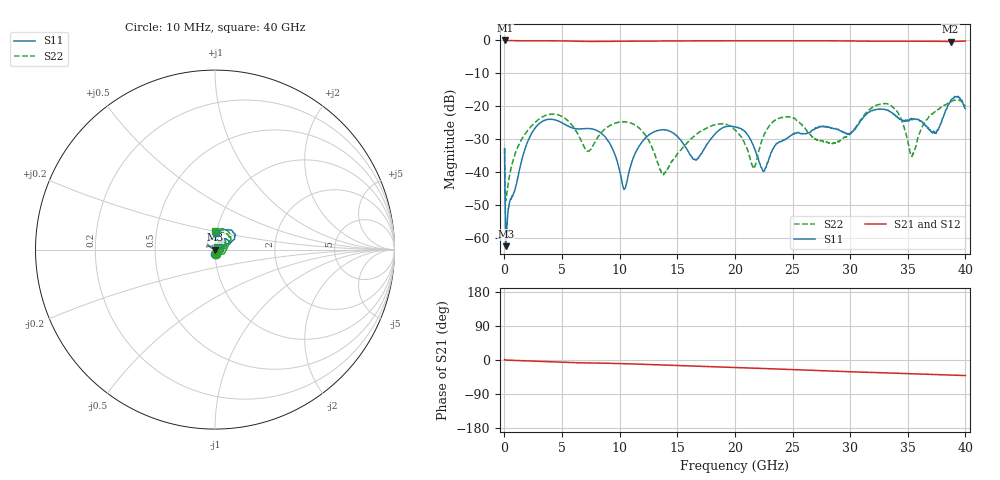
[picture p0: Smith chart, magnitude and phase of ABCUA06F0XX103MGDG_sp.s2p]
! Amotech Co.,Ltd.
! http://www.amotech.co.kr/
! Date: Wednesday, December 02, 2020 16:14:27
! Part Number: ABCUA 06F 0XX 103M GDG
! Freq. Start=10[MHz] Stop=40[GHz], 4000[Steps]
# Hz S  dB  R 50
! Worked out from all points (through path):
!   4000 points, 10 MHz to 40 GHz, reference 50 ohm
!   highest |S21| = -0.01 dB at 50 MHz (marker M1); lowest = -0.3 dB at 38.71 GHz (marker M2)
!   group delay of S21, straight-line fit = 2.85 ps
!   lowest |S11| = -62.4 dB at 140 MHz (marker M3), VSWR 1.00, Z = 49.9 + j0.0169 ohm
!   |S11| at or under -10 dB: start of sweep to end of sweep
!   |S22| runs from -48.5 to -18.0 dB; largest |S21 - S12| = 0.0046
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1e7  -32.76 -90.3  -0.02 1.3  -0.01 1.3  -32.72 -80.0
5e7  -47.88 -103.0  -0.01 0.2  -0.01 0.2  -45.68 -48.5
1.4e8  -62.35 167.2  -0.02 -0.2  -0.01 -0.2  -48.07 2.6
2.8e8  -52.97 97.8  -0.03 -0.5  -0.02 -0.5  -44.24 21.3
1.2e9  -40.93 145.3  -0.10 -1.6  -0.09 -1.5  -31.95 5.9
2.9e9  -25.57 142.3  -0.12 -3.2  -0.10 -3.2  -24.11 23.9
6.68e9  -26.78 22.5  -0.26 -7.4  -0.25 -7.4  -30.60 50.9
8.9e9  -29.97 -42.6  -0.29 -8.5  -0.27 -8.5  -26.33 -32.2
1.041e10  -44.95 -1.6  -0.23 -9.7  -0.22 -9.7  -24.69 -6.1
1.334e10  -27.29 -6.1  -0.15 -12.7  -0.13 -12.7  -37.41 104.8
1.655e10  -36.11 7.3  -0.13 -16.2  -0.11 -16.1  -28.82 -9.6
2.001e10  -26.24 31.6  -0.12 -19.8  -0.09 -19.7  -27.12 66.2
2.162e10  -32.12 17.7  -0.10 -21.5  -0.08 -21.4  -38.84 25.9
2.248e10  -39.57 56.3  -0.11 -22.5  -0.08 -22.4  -29.00 -23.0
2.452e10  -29.67 69.1  -0.11 -24.7  -0.09 -24.6  -23.15 18.4
2.667e10  -27.27 13.0  -0.11 -27.1  -0.09 -27.0  -29.05 65.2
2.888e10  -27.00 3.1  -0.14 -29.6  -0.11 -29.5  -30.75 47.4
3.334e10  -21.25 22.9  -0.24 -34.3  -0.22 -34.2  -19.41 61.9
3.538e10  -24.08 17.9  -0.24 -36.1  -0.22 -36.0  -35.09 41.5
3.734e10  -28.08 42.2  -0.26 -38.3  -0.24 -38.2  -21.65 20.1
3.871e10  -18.35 27.8  -0.34 -39.7  -0.31 -39.6  -18.60 43.7
4e10  -20.69 87.4  -0.19 -41.0  -0.17 -40.9  -19.97 90.3
